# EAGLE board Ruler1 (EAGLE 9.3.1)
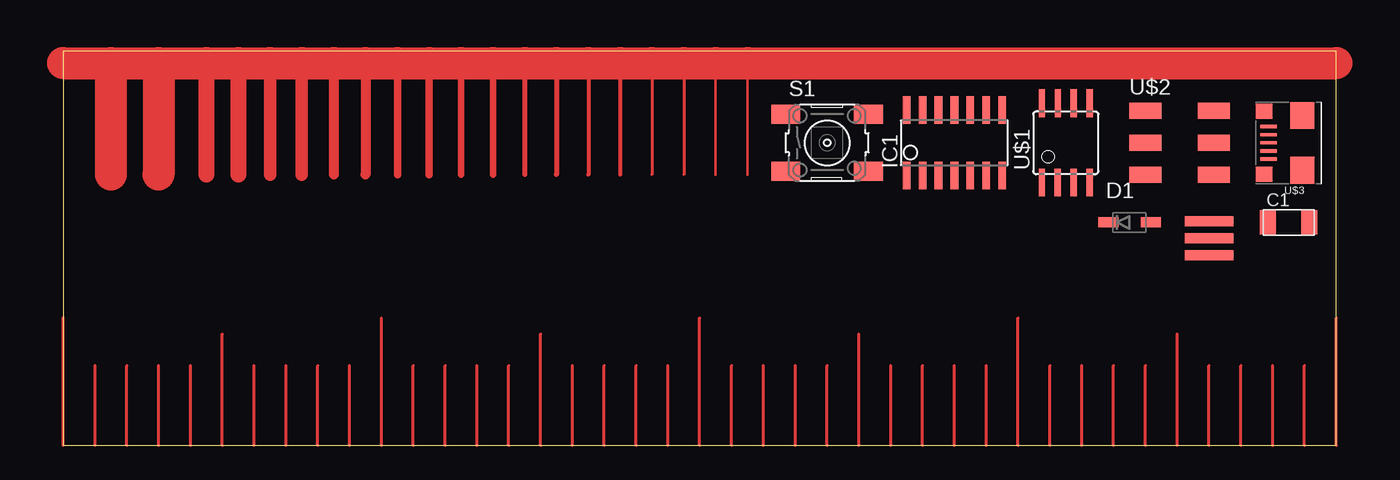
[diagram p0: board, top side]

Size 101.58 x 31.42 mm. Coordinates in mm from the lower left corner, seen from the top.
Outline: 0,0 101.58,0 101.58,31.42 0,31.42 0,0
Copper layers (1*16): Top 0.035mm / dielectric 1.5mm / Bottom 0.035mm
Design rules "default": minimum track width 6mil, minimum drill 0.35mm, track to track 6mil, track to pad 6mil, pad to pad 6mil, via to via 6mil, smd to smd 6mil, copper to edge 40mil, drill to drill 6mil, minimum pad ring 10mil, minimum via ring 8mil, stop-mask expansion 4mil, vias tented up to drill 0mil, thermal gap 10mil

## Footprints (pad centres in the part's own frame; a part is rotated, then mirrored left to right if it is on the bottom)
C1206FAB = smd 1.27 x 1.905: 1 -1.651,0; 2 1.651,0
SOD123 = smd 1.6 x 0.8: ANODE 1.7,0; CATHODE -1.7,0
SOIC14 = smd 0.61 x 2.21: 1 -3.81,-2.603; 2 -2.54,-2.603; 3 -1.27,-2.603; 4 0,-2.603; 5 1.27,-2.603; 6 2.54,-2.603; 7 3.81,-2.603; 8 3.81,2.603; 9 2.54,2.603; 10 1.27,2.603; 11 0,2.603; 12 -1.27,2.603; 13 -2.54,2.603; 14 -3.81,2.603
6MM_SWITCH = smd 2.286 x 1.524: 1 -3.302,2.286; 2 3.302,2.286; 3 -3.302,-2.286; 4 3.302,-2.286
SOIC8 = smd 0.5 x 2.2: 1 -1.905,-3.154; 2 -0.645,-3.154; 3 0.625,-3.154; 4 1.895,-3.154; 5 1.905,3.154; 6 0.635,3.154; 7 -0.635,3.154; 8 -1.905,3.154
2X03SMD = smd 2.54 x 1.27: 1 -2.54,2.54; 2 2.92,2.54; 3 -2.54,0; 4 2.92,0; 5 -2.54,-2.54; 6 2.92,-2.54
DX4R005HJ5_64 = smd 0.254 x 1.35: D+ 0,1.6; D- -0.65,1.6; GND 1.3,1.6; ID 0.65,1.6; VBUS -1.3,1.6 | smd 1.2 x 1.3: GND@1 -2.5,1.95; GND@2 2.5,1.95 | smd 2.15 x 1.9: GND@3 -2.175,-1.1; GND@4 2.175,-1.1
EFOBM = smd 0.8 x 3.9: 1 -1.35,0; 2 0,0; 3 1.35,0

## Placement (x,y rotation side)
C1  CAP-US1206FAB  [C1206FAB]  97.79,17.78 0 top
D1  [SOD123]  85.09,17.78 0 top
IC1  ATTINY44-SSU  [SOIC14]  71.12,24.13 0 top
S1  [6MM_SWITCH]  60.96,24.13 0 top
U$1  ATTINY45SI  [SOIC8]  80.01,24.13 0 top
U$2  AVRISPSMD  [2X03SMD]  88.9,24.13 0 top
U$3  MICRO-USB_1/64  [DX4R005HJ5_64]  97.79,24.13 90 top
U$4  RESONATOR  [EFOBM]  91.44,16.51 90 top

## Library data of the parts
C1 D1 IC1 S1 U$1-U$4 = Fab_Lib

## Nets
GND: IC1.14
VCC: IC1.1

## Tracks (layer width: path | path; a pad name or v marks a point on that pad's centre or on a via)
N$1
  Top 0.203: 52.07,30.48 52.07,21.59 | 54.61,30.48 54.61,21.59
  Top 0.254: 46.99,30.48 46.99,21.59 | 49.53,30.48 49.53,21.59
  Top 0.305: 41.91,30.48 41.91,21.59 | 44.45,30.48 44.45,21.59
  Top 0.406: 36.83,30.48 36.83,21.59 | 39.37,30.48 39.37,21.59
  Top 0.508: 31.75,30.48 31.75,21.59 | 34.29,30.48 34.29,21.59
  Top 0.61: 26.67,30.48 26.67,21.59 | 29.21,30.48 29.21,21.59
  Top 0.813: 21.59,30.48 21.59,21.59 | 24.13,30.48 24.13,21.59
  Top 1.016: 16.51,30.48 16.51,21.59 | 19.05,30.48 19.05,21.59
  Top 1.27: 11.43,30.48 11.43,21.59 | 13.97,30.48 13.97,21.59
  Top 2.54: 0,30.48 3.81,30.48 | 3.81,30.48 7.62,30.48 | 7.62,30.48 11.43,30.48 13.97,30.48 16.51,30.48 19.05,30.48 21.59,30.48 24.13,30.48 26.67,30.48 29.21,30.48 31.75,30.48 34.29,30.48 36.83,30.48 39.37,30.48 41.91,30.48 44.45,30.48 46.99,30.48 49.53,30.48 52.07,30.48 54.61,30.48 101.6,30.48 | 3.81,30.48 3.81,21.59 | 7.62,30.48 7.62,21.59
N$2
  Top 0.254: 0,0 0,10.16
N$3
  Top 0.254: 2.54,0 2.54,6.35
N$4
  Top 0.254: 5.08,0 5.08,6.35
N$5
  Top 0.254: 7.62,0 7.62,6.35
N$6
  Top 0.254: 10.16,0 10.16,6.35
N$7
  Top 0.254: 12.7,0 12.7,8.89
N$8
  Top 0.254: 15.24,0 15.24,6.35
N$9
  Top 0.254: 17.78,0 17.78,6.35
N$10
  Top 0.254: 20.32,0 20.32,6.35
N$11
  Top 0.254: 22.86,0 22.86,6.35
N$12
  Top 0.254: 25.4,0 25.4,10.16
N$13
  Top 0.254: 27.94,0 27.94,6.35
N$14
  Top 0.254: 30.48,0 30.48,6.35
N$15
  Top 0.254: 33.02,0 33.02,6.35
N$16
  Top 0.254: 35.56,0 35.56,6.35
N$17
  Top 0.254: 38.1,0 38.1,8.89
N$18
  Top 0.254: 40.64,0 40.64,6.35
N$19
  Top 0.254: 43.18,0 43.18,6.35
N$20
  Top 0.254: 45.72,0 45.72,6.35
N$21
  Top 0.254: 48.26,0 48.26,6.35
N$22
  Top 0.254: 50.8,0 50.8,10.16
N$23
  Top 0.254: 53.34,0 53.34,6.35
N$24
  Top 0.254: 55.88,0 55.88,6.35
N$25
  Top 0.254: 58.42,0 58.42,6.35
N$26
  Top 0.254: 60.96,0 60.96,6.35
N$27
  Top 0.254: 63.5,0 63.5,8.89
N$28
  Top 0.254: 66.04,0 66.04,6.35
N$29
  Top 0.254: 68.58,0 68.58,6.35
N$30
  Top 0.254: 71.12,0 71.12,6.35
N$31
  Top 0.254: 73.66,0 73.66,6.35
N$32
  Top 0.254: 76.2,0 76.2,10.16
N$33
  Top 0.254: 78.74,0 78.74,6.35
N$34
  Top 0.254: 81.28,0 81.28,6.35
N$35
  Top 0.254: 83.82,0 83.82,6.35
N$36
  Top 0.254: 86.36,0 86.36,6.35
N$37
  Top 0.254: 88.9,0 88.9,8.89
N$38
  Top 0.254: 91.44,0 91.44,6.35
N$39
  Top 0.254: 93.98,0 93.98,6.35
N$40
  Top 0.254: 96.52,0 96.52,6.35
N$41
  Top 0.254: 99.06,0 99.06,6.35
N$42
  Top 0.254: 101.6,0 101.6,10.16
